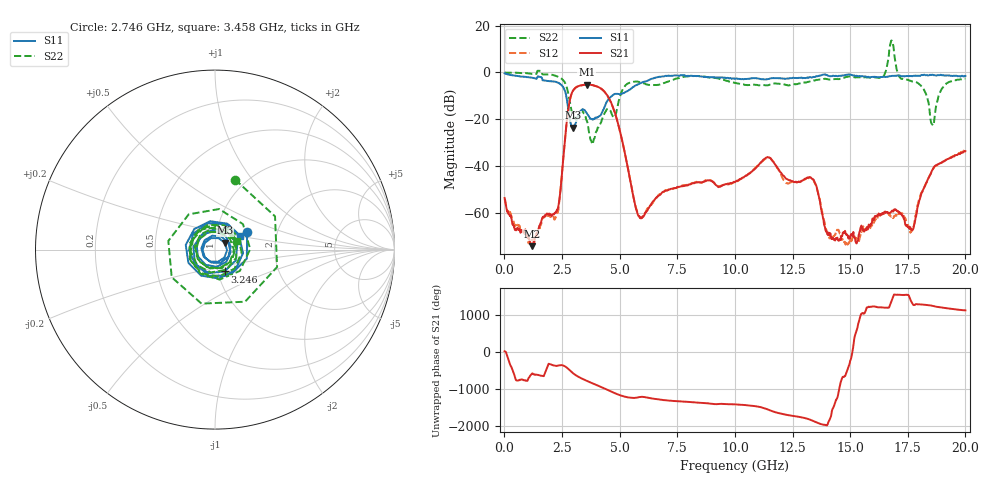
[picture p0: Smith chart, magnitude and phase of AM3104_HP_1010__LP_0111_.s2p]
!Created with skrf (http://scikit-rf.org).
# Hz S RI R 50.0
!freq ReS11 ImS11 ReS21 ImS21 ReS12 ImS12 ReS22 ImS22
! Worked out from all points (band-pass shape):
!   1601 points, 10 MHz to 20 GHz, reference 50 ohm
!   highest |S21| = -5.15 dB at 3.571 GHz (marker M1); lowest = -73.9 dB at 1.184 GHz (marker M2)
!   |S21| within 3 dB of the highest: 2.954 GHz to 4.341 GHz (1.387 GHz wide, 38 % of centre)
!   lowest |S11| = -23.5 dB at 2.971 GHz (marker M3), VSWR 1.14, Z = 55.6 + j4.27 ohm
!   |S11| at or under -10 dB: 2.684 GHz to 4.66 GHz (1.976 GHz wide, 53.8 % of centre)
!   |S22| runs from -30.6 to 13.6 dB; largest |S21 - S12| = 0.036
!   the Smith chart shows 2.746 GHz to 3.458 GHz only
!   S11 on the Smith chart (normalised r, x): 2.746 GHz: 1.40, +0.29; 3.246 GHz: 1.08, -0.27; 3.458 GHz: 1.31, +0.21
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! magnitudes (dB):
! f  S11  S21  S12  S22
! 10 MHz  -0.4  -53.4  -53.9  0.0
! 1.184 GHz  -2.2  -73.9  -71.5  -0.6
! 2.271 GHz  -4.1  -58.7  -60.8  -1.6
! 2.746 GHz  -13.8  -17.6  -17.6  -7.8
! 2.971 GHz  -23.5  -7.8  -7.8  -18.5
! 3.246 GHz  -17.5  -5.6  -5.7  -17.8
! 3.346 GHz  -16.0  -5.4  -5.5  -16.5
! 3.458 GHz  -15.9  -5.2  -5.3  -17.5
! 3.571 GHz  -17.3  -5.1  -5.2  -20.5
! 3.821 GHz  -20.0  -5.3  -5.4  -30.6
! 4.683 GHz  -9.8  -14.0  -14.2  -18.2
! 5.845 GHz  -4.9  -61.2  -61.0  -4.0
! 6.682 GHz  -1.9  -52.6  -52.2  -5.2
! 10.01 GHz  -2.7  -46.7  -46.8  -4.5
! 11.44 GHz  -2.8  -36.1  -36.2  -5.4
! 13.34 GHz  -2.1  -45.2  -45.2  -3.7
! 14.28 GHz  -1.4  -70.8  -69.6  -2.8
! 16.68 GHz  -1.6  -59.9  -60.3  7.2
! 17.68 GHz  -1.6  -67.0  -66.9  -3.8
! 18.56 GHz  -0.9  -41.6  -41.6  -22.2
! 19.03 GHz  -1.2  -38.0  -37.9  -6.3
! 20 GHz  -1.5  -33.5  -32.9  -2.5
